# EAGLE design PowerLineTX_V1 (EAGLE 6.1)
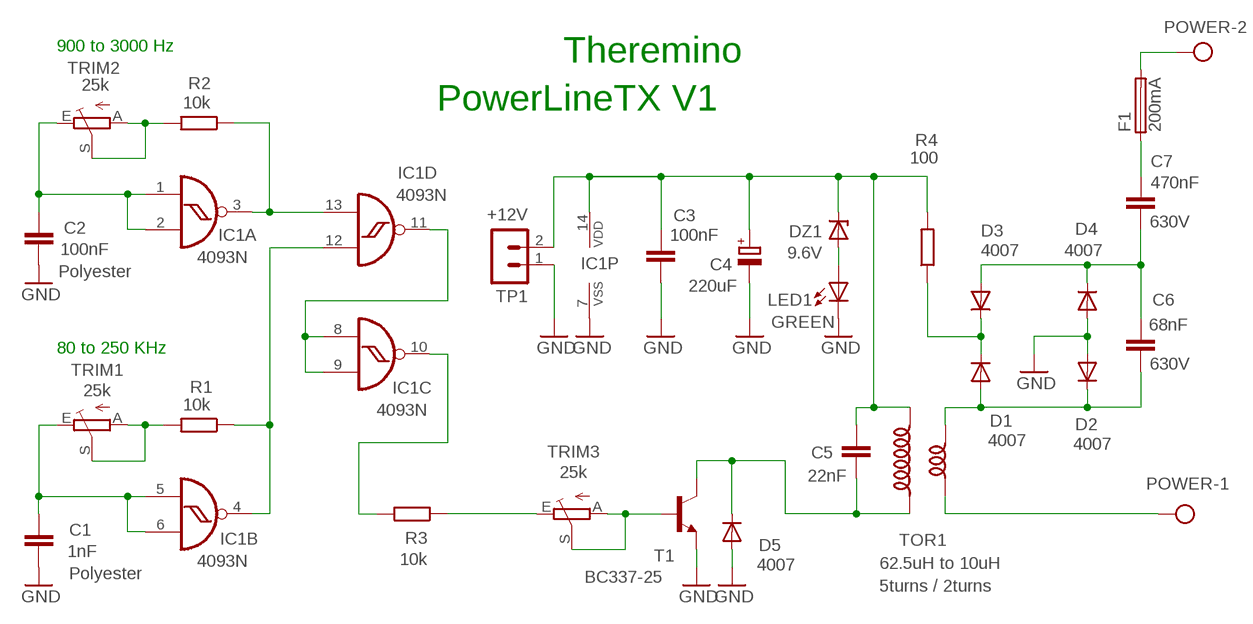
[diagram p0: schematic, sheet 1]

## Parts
C1  1nF  C5/2.5  [C5B2.5]
C2  100nF  C5/2.5  [C5B2.5]
C3  100nF  C5/2.5  [C5B2.5]
C4  220uF  CPOL-EUE5-8.5  [E5-8,5]
C5  22nF  C7.5/3  [C7.5B3]
C6  68nF  C15/5  [C15B5]
C7  470nF  C22/7  [C22.5B7]
D1  4007  DIODE-DO35-10  [DO35-10]
D2  4007  DIODE-DO35-10  [DO35-10]
D3  4007  DIODE-DO35-10  [DO35-10]
D4  4007  DIODE-DO35-10  [DO35-10]
D5  4007  DIODE-DO35-10  [DO35-10]
DZ1  9.6V  ZENER-DIODEDO34-7  [DO34Z7]
F1  200mA  FUSE_22,5  [FUSE_22,5]
IC1  4093N  [DIL14]
LED1  GREEN  LED3MM_F  [LED3MM]
POWER  AK500/2  [AK500/2]
R1  10k  R-EU_0207/10  [0207/10]
R2  10k  R-EU_0207/10  [0207/10]
R3  10k  R-EU_0207/10  [0207/10]
R4  100  R-EU_0207/12  [0207/12]
T1  BC337-25  -NPN-TO92-CBE  [TO92-CBE]
TOR1  62.5uH to 10uH  INDUCTOR_DUALTOR2B  [TOROID_2B]
TP1  +12V  MA02-1L2  [MA02-1_L2]
TRIM1  25k  TRIMMERTRIM_M1  [TRIM_M1]
TRIM2  25k  TRIMMERTRIM_M1  [TRIM_M1]
TRIM3  25k  TRIMMERTRIM_2H  [TRIM_2H]

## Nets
GND: C1.2 C2.2 C3.2 C4.V- D2.A D4.A D5.A IC1.7(P:VSS) LED1.K(C) T1.E TP1.1
N$2: C6.2 C7.1 D3.A D4.C
N$3: C7.2 F1.1
N$4: D1.C D3.C R4.1
N$5: C6.1 D1.A D2.C TOR1.3
N$6: IC1.3(A:O) IC1.13(D:I1) R2.1
N$7: POWER.1 TOR1.4
N$8: F1.2 POWER.2
N$9: IC1.4(B:O) IC1.12(D:I0) R1.1
N$10: C3.1 C4.V+ C5.2 DZ1.C IC1.14(P:VDD) R4.2 TOR1.1 TP1.2
N$11: R1.2 TRIM1.A TRIM1.S
N$12: C2.1 IC1.1(A:I0) IC1.2(A:I1) TRIM2.E
N$13: C1.1 IC1.5(B:I0) IC1.6(B:I1) TRIM1.E
N$14: R2.2 TRIM2.A TRIM2.S
N$15: R3.1 TRIM3.E
N$16: C5.1 D5.C T1.C TOR1.2
N$17: IC1.8(C:I0) IC1.9(C:I1) IC1.11(D:O)
N$18: T1.B TRIM3.A TRIM3.S
N$19: IC1.10(C:O) R3.2
N$20: DZ1.A LED1.A

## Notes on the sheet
- 900 to 3000 Hz
- Theremino
- PowerLineTX V1
- 80 to 250 KHz

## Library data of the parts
C1 C2 = 00-LIVIO:C: CAPACITOR; 1: Polyester
C3 = 00-LIVIO:C: CAPACITOR
C4 = 00-LIVIO:CPOL-EU: POLARIZED CAPACITOR, European symbol
C5 = capacitor-wima:C: CAPACITOR
C6 C7 = capacitor-wima:C: CAPACITOR; 1: 630V
D1-D5 = 00-LIVIO:DIODE-: DIODE
DZ1 = 00-LIVIO:ZENER-DIODE: Z-Diode
F1 = 00-LIVIO:FUSE_22,5: FUSE HOLDER
IC1 = 40xx:4093: Quad 2-input NAND schmitt trigger
LED1 = 00-LIVIO:LED: LEDS
POWER = 07-con-ptr500:AK500/2: CONNECTOR
R1-R4 = 00-LIVIO:R-EU_: RESISTOR, European symbol
T1 = 00-LIVIO:*-NPN-: NPN Transistror
TOR1 = 00-LIVIO:INDUCTOR_DUAL; 1: 5turns / 2turns
TP1 = 03-con-lstb-M:MA02-1: PIN HEADER
TRIM1-TRIM3 = 00-LIVIO:TRIMMER: Horizzontal and Vertical trimmers

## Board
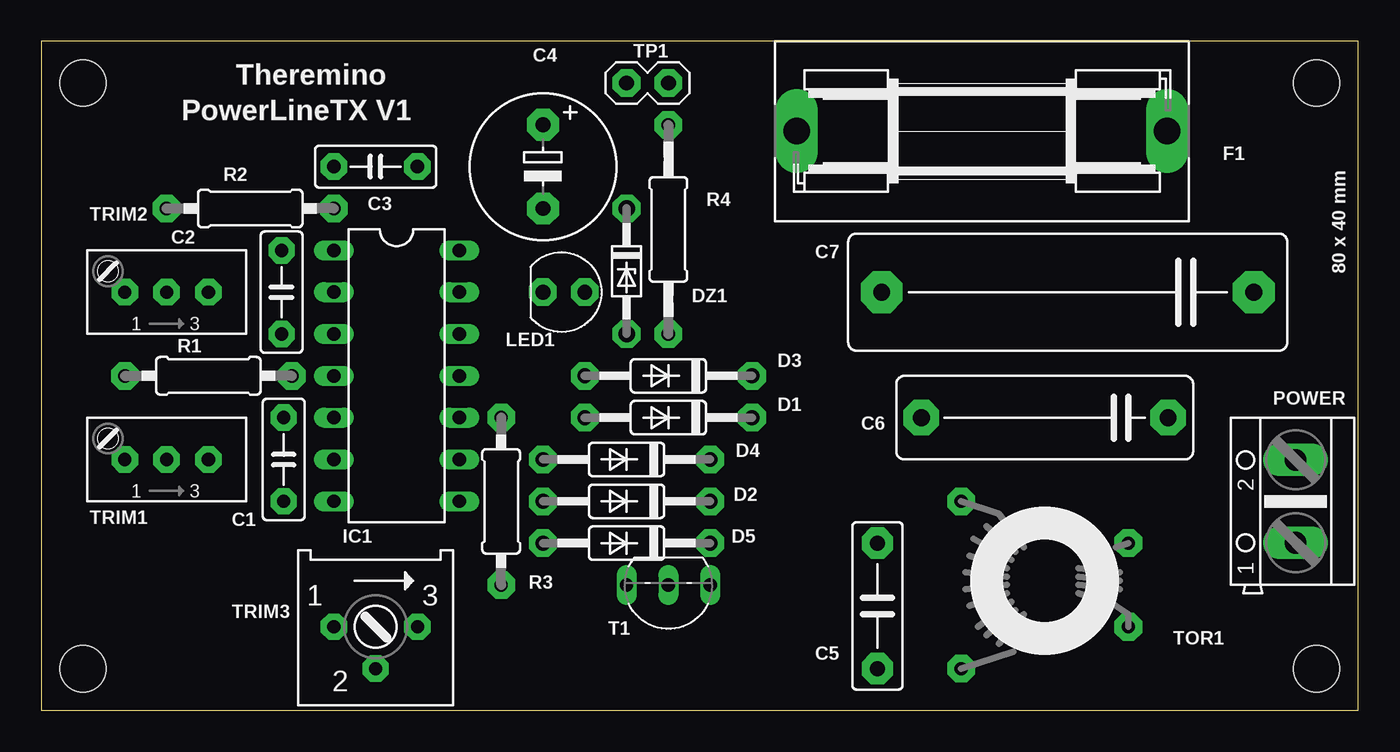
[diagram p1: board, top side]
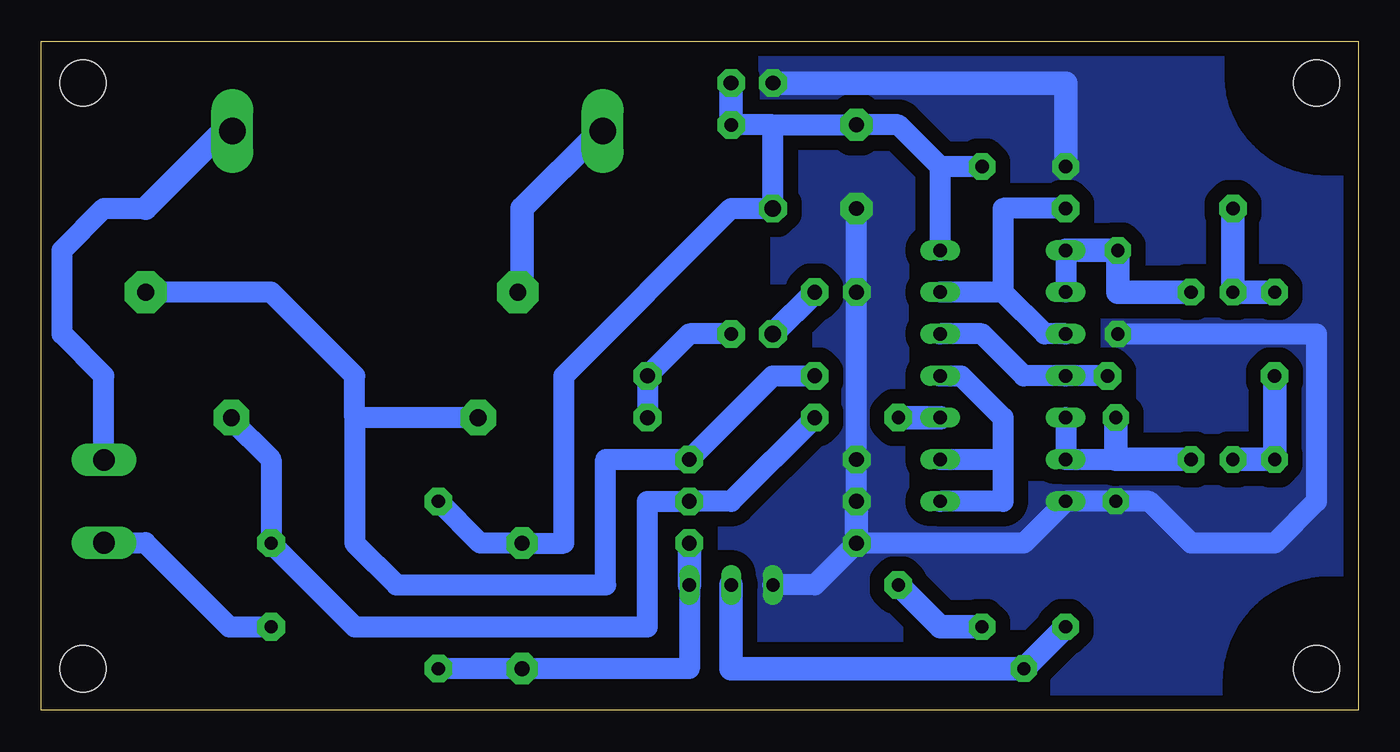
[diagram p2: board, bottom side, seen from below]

Size 80.01 x 40.64 mm. Coordinates in mm from the lower left corner, seen from the top.
Outline: 80.01,40.64 0,40.64 0,0 80.01,0 80.01,40.64
Copper layers (1*16): Top 0.035mm / dielectric 1.5mm / Bottom 0.035mm
Design rules: minimum track width 10mil, minimum drill 31mil, track to track 31mil, track to pad 31mil, pad to pad 31mil, via to via 31mil, smd to smd 31mil, copper to edge 31mil, drill to drill 8mil, minimum pad ring 5mil, minimum via ring 8mil, stop-mask expansion 4mil, vias tented up to drill 0mil, thermal gap 47mil
Holes 2.8 mm at 2.54,2.54 2.54,38.1 77.47,2.54 77.47,38.1
bRestrict: 3 lines

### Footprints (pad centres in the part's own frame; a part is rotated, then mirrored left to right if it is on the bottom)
C5B2.5 = drill 0.813 pad 1.6 octagon: 1 -2.54,0; 2 2.54,0
E5-8,5 = drill 0.9 pad 1.93 octagon: V+ -2.54,0; V- 2.54,0
C7.5B3 = drill 0.914 pad 1.905 octagon: 1 -3.81,0; 2 3.81,0
C15B5 = drill 1.016 pad 2.159 octagon: 1 -7.493,0; 2 7.493,0
C22.5B7 = drill 1.016 pad 2.54 octagon: 1 -11.303,0; 2 11.303,0
DO35-10 = drill 0.9 pad 1.676 octagon: A 5.08,0; C -5.08,0
DO34Z7 = drill 1 pad 1.676 octagon: A 3.81,0; C -3.81,0
FUSE_22,5 = drill 1.6 pad 2.54 long: 1 -11.252,0; 2 11.252,0
DIL14 = drill 0.813 long: 1 -7.62,-3.81; 2 -5.08,-3.81; 3 -2.54,-3.81; 4 0,-3.81; 5 2.54,-3.81; 6 5.08,-3.81; 7 7.62,-3.81; 8 7.62,3.81; 9 5.08,3.81; 10 2.54,3.81; 11 0,3.81; 12 -2.54,3.81; 13 -5.08,3.81; 14 -7.62,3.81
LED3MM = drill 0.9 pad 1.676 octagon: A -1.27,0; K 1.27,0
AK500/2 = drill 1.321 long: 1 -2.515,0; 2 2.515,0
0207/10 = drill 0.813 pad 1.676 octagon: 1 -5.08,0; 2 5.08,0
0207/12 = drill 0.813 pad 1.676 octagon: 1 -6.35,0; 2 6.35,0
TO92-CBE = drill 0.813 long: B 0,0; C -2.54,0; E 2.54,0
TOROID_2B = drill 0.8 pad 1.676 octagon: 1 -5.08,5.08; 2 -5.08,-5.08; 3 5.08,2.54; 4 5.08,-2.54
MA02-1_L2 = drill 0.9 pad 1.676 octagon: 1 -1.27,0; 2 1.27,0
TRIM_M1 = drill 0.8 pad 1.6 octagon: A 2.54,0; E -2.54,0; S 0,0
TRIM_2H = drill 0.8 pad 1.6 octagon: A 2.54,0; E -2.54,0; S 0,2.54

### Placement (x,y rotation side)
C1  14.73,15.24 270 top
C2  14.61,25.4 270 top
C3  20.32,33.02 180 top
C4  30.48,33.02 270 top
C5  50.8,6.35 90 top
C6  60.96,17.78 180 top
C7  62.36,25.4 180 top
D1  38.1,17.78 180 top
D2  35.56,12.7 180 top
D3  38.1,20.32 180 top
D4  35.56,15.24 180 top
D5  35.56,10.16 180 top
DZ1  35.56,26.67 270 top
F1  57.15,35.18 0 top
IC1  21.59,20.32 270 top
LED1  31.75,25.4 180 top
POWER  76.2,12.7 90 top
R1  10.16,20.32 180 top
R2  12.7,30.48 180 top
R3  27.94,12.7 90 top
R4  38.1,29.21 90 top
T1  38.1,7.62 180 top
TOR1  60.96,7.62 0 top
TP1  36.83,38.1 0 top
TRIM1  7.62,15.24 180 top
TRIM2  7.62,25.4 180 top
TRIM3  20.32,5.08 180 top

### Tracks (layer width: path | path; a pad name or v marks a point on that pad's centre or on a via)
GND
  Bottom 1.27: C4.V- D4.A D2.A | C2.2 2.54,22.86 2.54,12.7 5.08,10.16 10.16,10.16 12.7,12.7 C1.2 IC1.7 20.32,10.16 D5.A 33.02,7.62 T1.E
  Bottom 1.422: D5.A D2.A | TP1.1 17.78,38.1 C3.2
  pour Bottom (isolate 0.9, rank 6, no thermals): -1,-1 81.01,-1 81.01,41.64 -1,41.64
N$2
  Bottom 1.27: D3.A 35.56,20.32 D4.C 45.72,15.24 45.72,7.62 58.42,7.62 60.96,10.16 60.96,17.78 | 60.96,17.78 60.96,20.32 66.04,25.4 C7.1 | C6.2 60.96,17.78
N$3
  Bottom 1.422: C7.2 50.8,25.4 50.8,30.48 46.1,35.18 F1.1
N$4
  Bottom 1.27: R4.1 40.64,22.86 D3.C D1.C
N$5
  Bottom 1.27: D1.A 38.1,12.7 D2.C 43.18,12.7 43.18,5.08 60.96,5.08 TOR1.3 66.04,15.24 68.58,17.78 C6.1
N$6
  Bottom 1.27: IC1.3 19.05,22.86 21.59,25.4 | 21.59,25.4 IC1.13 | R2.1 21.59,30.48 21.59,25.4
N$7
  Bottom 1.27: POWER.1 73.69,10.19 68.58,5.08 TOR1.4
N$8
  Bottom 1.27: POWER.2 76.2,20.32 78.74,22.86 78.74,27.94 76.2,30.48 73.66,30.48
  Bottom 1.422: F1.2 68.58,35.36 | 68.58,35.36 68.58,35.56 | 68.58,35.56 68.58,35.36 | 68.58,35.36 68.58,35.56 | 68.58,35.56 | 68.58,35.56 73.66,30.48
N$9
  Bottom 1.27: IC1.12 22.86,22.86 20.32,20.32 IC1.4 R1.1
N$10
  Bottom 1.27: IC1.14 25.4,33.02 | C3.1 25.4,33.02 | 25.4,33.02 27.94,35.56 C4.V+ 35.56,35.56 | 35.56,35.56 DZ1.C 38.1,30.48 48.26,20.32 48.26,10.16 C5.2 53.34,10.16 TOR1.1 | 35.56,35.56 R4.2
  Bottom 1.422: R4.2 TP1.2
N$11
  Bottom 1.422: TRIM1.S TRIM1.A R1.2
N$12
  Bottom 1.27: IC1.1 IC1.2
  Bottom 1.422: TRIM2.E 12.7,25.4 14.61,25.4 C2.1 IC1.1
N$13
  Bottom 1.27: IC1.5 IC1.6 14.73,15.24
  Bottom 1.422: TRIM1.E 14.73,15.24 C1.1
N$14
  Bottom 1.422: TRIM2.A TRIM2.S R2.2
N$15
  Bottom 1.422: TRIM3.E 25.4,5.08 R3.1
N$16
  Bottom 1.27: T1.C 40.64,2.54 C5.1 TOR1.2
  Bottom 1.422: D5.C T1.C
N$17
  Bottom 1.27: IC1.11 24.13,20.32 21.59,17.78 21.59,15.24 | 21.59,15.24 21.59,12.7 IC1.8 | IC1.9 21.59,15.24
N$18
  Bottom 1.422: T1.B 38.1,2.54 TRIM3.S TRIM3.A
N$19
  Bottom 1.422: IC1.10 R3.2
N$20
  Bottom 1.422: DZ1.A LED1.A

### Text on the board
tNames: Theremino | PowerLineTX V1 | 80 x 40 mm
